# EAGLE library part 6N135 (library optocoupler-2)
MOTOROLA OPTO COUPLER
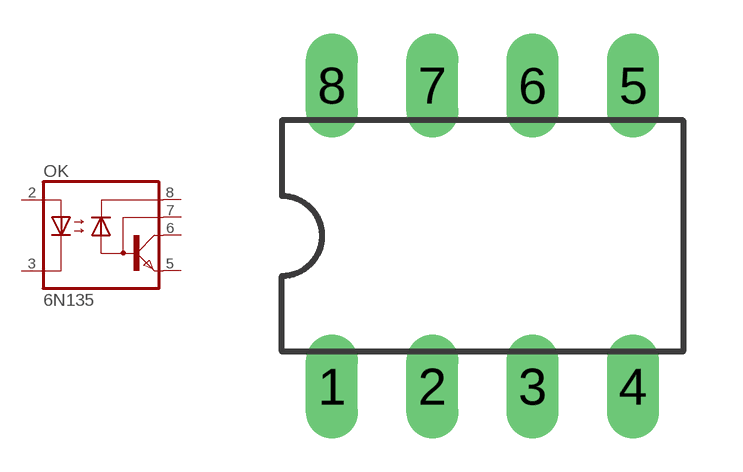
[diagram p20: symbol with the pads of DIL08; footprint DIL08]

Designator prefix OK

## 6N135  [DIL08]
2  A  pas
3  C  pas
5  GND  pas
6  VO  pas
7  VB  pas
8  VCC  pas

## Footprint DIL08 (pad centres in mm)
Dual In Line Package
drill 0.813 long: 1 -3.81,-3.81; 2 -1.27,-3.81; 3 1.27,-3.81; 4 3.81,-3.81; 5 3.81,3.81; 6 1.27,3.81; 7 -1.27,3.81; 8 -3.81,3.81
